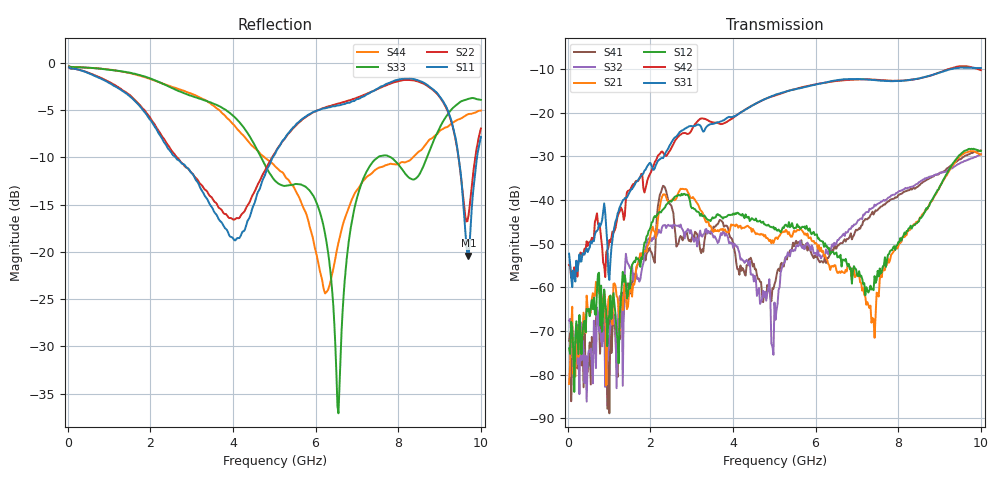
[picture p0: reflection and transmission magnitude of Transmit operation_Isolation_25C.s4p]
! Device:  ADRF5545A
! Description: Dual-Channel, Receiver Front End
! Frequency:  2.4 -  4.2 GHz
! Ports:
!	ANT-CHA	= Port 1
!	ANT-CHB	= Port 2
!  TXOUT-CHA = Port 3
!	TXOUT-CHB = Port 4
! VDD1-CHA, VDD1-CHB, VDD2-CHA, VDD2-CHB, and SWVDD-CHAB = 5 V
! SWCTRL-CHAB = 0 V,  PD-CHAB = 0 V,BP-CHA=BP-CHB=0V
! Temp=25C
! Data:  Data was collected using a calibrated 4 port network analyzer and de-embedded using AtaiTec's In Situ De-Embedding.
! Note:  Analog Devices supplies this data as a sample of measured data
!  for this product.  Your particular data for this product may vary.
!  Data was taken at 25 degrees C.
!  Analog Devices reserves the right to change this data at anytime.
!Correction: S11(Full 4 Port(1,2,3,4))
!S12(Full 4 Port(1,2,3,4))
!S13(Full 4 Port(1,2,3,4))
!S14(Full 4 Port(1,2,3,4))
!S21(Full 4 Port(1,2,3,4))
!S22(Full 4 Port(1,2,3,4))
!S23(Full 4 Port(1,2,3,4))
!S24(Full 4 Port(1,2,3,4))
!S31(Full 4 Port(1,2,3,4))
!S32(Full 4 Port(1,2,3,4))
!S33(Full 4 Port(1,2,3,4))
!S34(Full 4 Port(1,2,3,4))
!S41(Full 4 Port(1,2,3,4))
!S42(Full 4 Port(1,2,3,4))
!S43(Full 4 Port(1,2,3,4))
!S44(Full 4 Port(1,2,3,4))
!S4P File: Measurements: <S11,S12,S13,S14>,
!<S21,S22,S23,S24>,
!<S31,S32,S33,S34>,
!<S41,S42,S43,S44>:
# Hz S  dB  R 50
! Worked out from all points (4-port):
!   400 points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, 34.98 MHz to 10 GHz, reference 50 ohm
!   strongest paths, dB at 34.98 MHz, 2.532 GHz, 5.03 GHz, 7.527 GHz, 10 GHz:
!     S31: -52.3, -26.4, -15.8, -12.6, -9.7
!     S42: -54.9, -27.6, -16.0, -12.5, -10.2
!     S12: -74.0, -40.0, -46.4, -57.5, -28.8
!     S21: -82.2, -39.8, -48.6, -62.1, -29.5
!     S32: -67.6, -46.5, -67.5, -40.8, -29.5
!     S41: -72.3, -42.1, -58.6, -41.9, -28.6
!   lowest |S11| = -20.4 dB at 9.7 GHz (marker M1), VSWR 1.21, Z = 41.7 + j2.65 ohm
!   |S11| at or under -10 dB: 2.609 GHz to 4.966 GHz (2.356 GHz wide, 62.2 % of centre); 9.46 GHz to 9.907 GHz (447.4 MHz wide, 4.62 % of centre)
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3.4975e7  -0.48 -10.3  -74.00 -119.6  -52.60 -7.2  -62.07 11.0
          -82.15 72.1  -0.53 -10.2  -69.27 -123.5  -51.54 -25.2
          -52.29 -6.6  -67.62 78.1  -0.39 -5.7  -74.77 114.5
          -72.25 -4.9  -54.87 -20.4  -67.83 49.5  -0.36 -5.7
1.2088e9  -2.65 -91.3  -72.00 148.0  -42.03 108.9  -79.24 -49.6
          -62.34 -166.2  -2.55 -90.5  -76.32 124.7  -42.20 107.9
          -43.06 142.9  -69.79 62.8  -0.85 -46.5  -82.09 66.5
          -80.57 65.1  -43.72 132.5  -73.92 -112.3  -0.85 -44.1
2.3077e9  -8.24 -172.4  -42.14 133.6  -30.16 100.3  -67.61 90.9
          -38.73 140.5  -7.93 -170.8  -65.46 107.8  -30.26 102.1
          -30.38 117.2  -45.80 -172.5  -2.23 -84.6  -74.33 178.9
          -36.72 -166.9  -29.06 109.8  -80.05 118.7  -2.22 -85.7
4.980025e9  -9.90 42.8  -46.10 -37.9  -15.57 30.7  -60.20 50.5
            -49.85 -20.8  -9.78 45.8  -59.55 36.3  -15.60 34.2
            -16.00 32.2  -75.47 140.5  -12.28 156.7  -68.53 138.4
            -60.33 108.5  -16.16 34.5  -73.11 147.9  -10.74 154.0
6.55345e9  -4.50 63.6  -52.90 -105.4  -12.52 -28.8  -48.52 -23.6
           -56.67 -72.9  -4.31 66.1  -51.16 -27.4  -12.66 -25.2
           -12.44 -27.6  -49.14 -11.4  -37.08 2.5  -44.07 142.9
           -50.41 -31.3  -12.63 -23.6  -44.82 139.5  -19.03 -18.2
9.7003e9  -20.42 160.7  -28.28 -112.5  -9.65 -151.2  -29.62 65.5
          -28.85 -120.4  -16.16 160.3  -31.90 60.8  -9.30 -145.5
          -9.64 -151.8  -30.64 67.9  -3.81 -159.6  -31.15 -143.3
          -29.49 66.6  -9.38 -146.4  -31.16 -145.5  -5.42 -148.4
1e10  -7.84 -149.7  -28.77 -162.2  -9.69 -175.2  -28.90 29.5
      -29.51 -170.0  -6.96 -161.6  -31.01 28.9  -10.07 -172.9
      -9.72 -175.9  -29.46 34.5  -3.92 -149.0  -28.47 -155.8
      -28.59 28.4  -10.20 -173.6  -28.84 -158.8  -5.06 -143.5
